PROGRAM LadderLogicExample
VAR_INPUT
	TOGGLE_RUN_ENABLE : BOOL;
	SETPOINT_PERCENT : UINT;
END_VAR
VAR_OUTPUT
	AC_LINE_VOLTAGE : UINT;
END_VAR
VAR
END_VAR

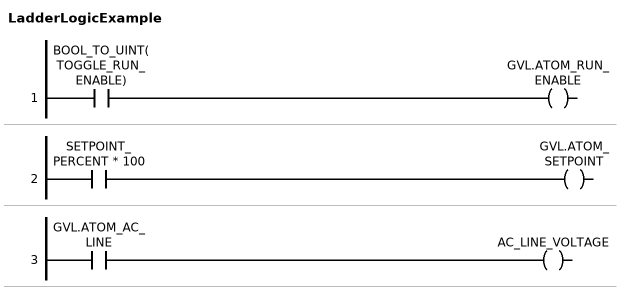
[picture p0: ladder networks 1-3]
// NETWORK 1
GVL.ATOM_RUN_ENABLE := BOOL_TO_UINT(TOGGLE_RUN_ENABLE);

// NETWORK 2
GVL.ATOM_SETPOINT := SETPOINT_PERCENT * 100;

// NETWORK 3
AC_LINE_VOLTAGE := GVL.ATOM_AC_LINE;

END_PROGRAM
